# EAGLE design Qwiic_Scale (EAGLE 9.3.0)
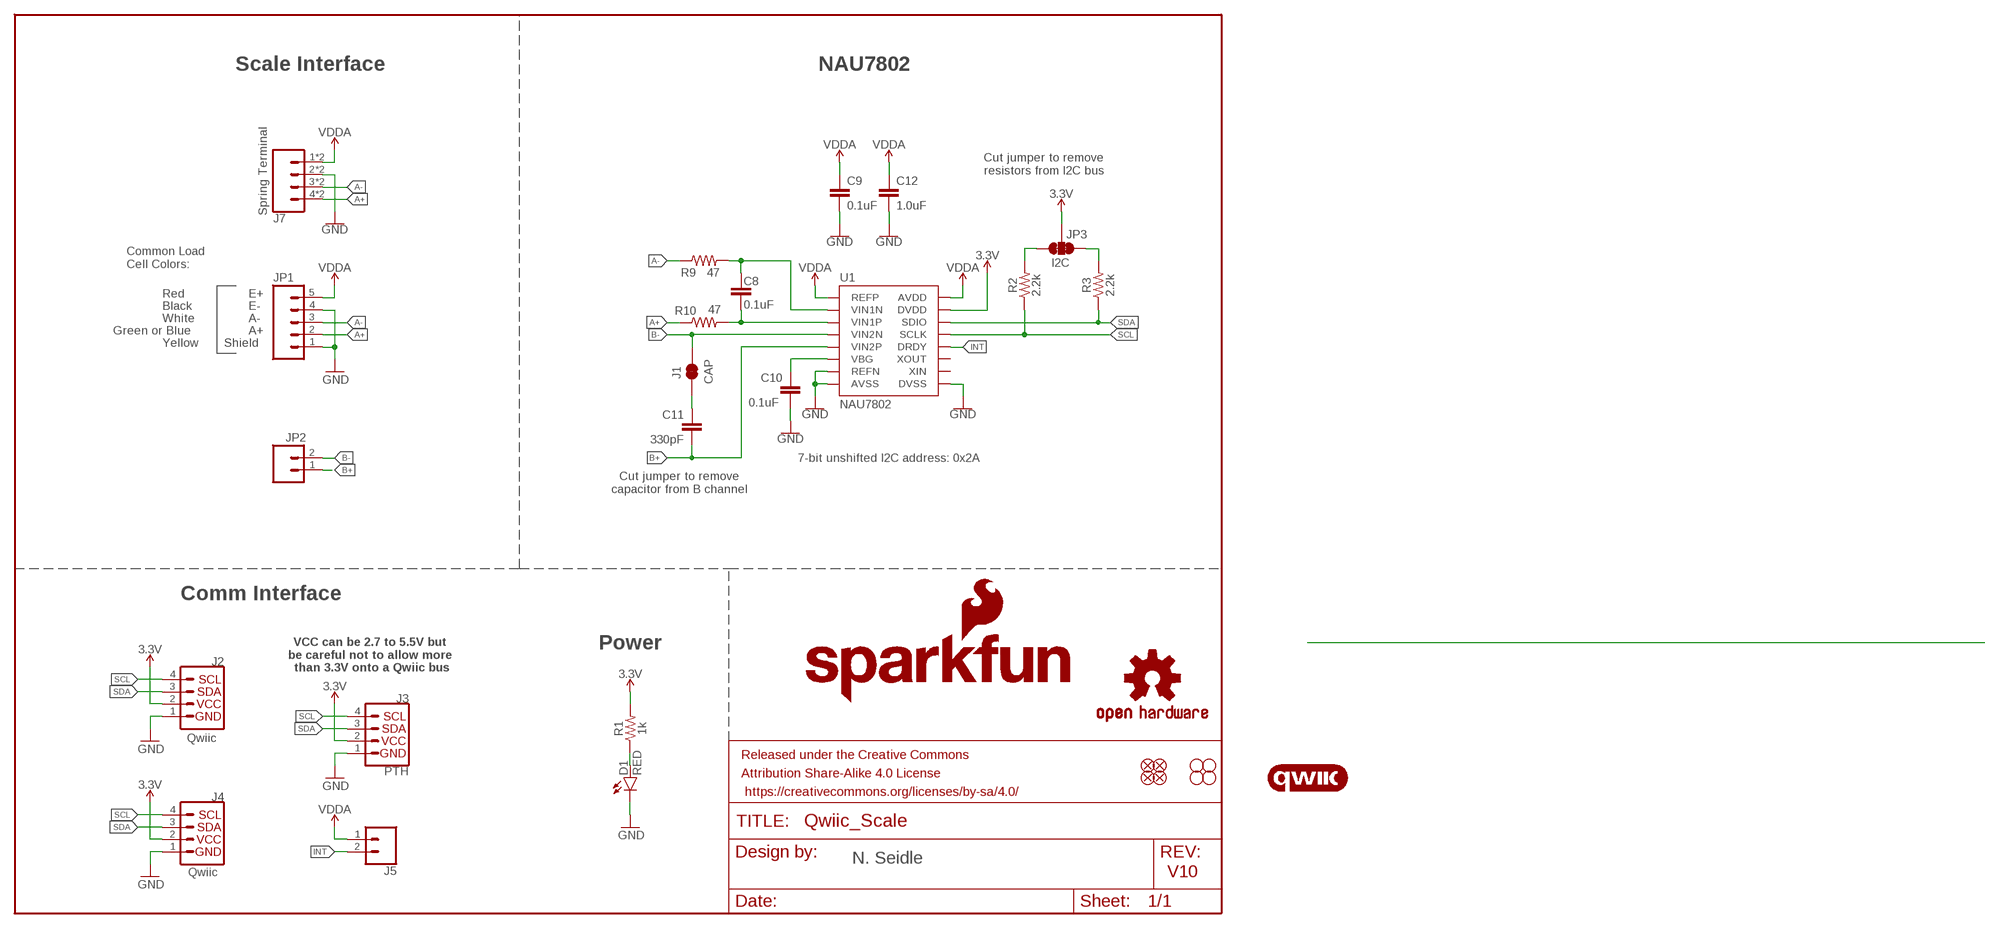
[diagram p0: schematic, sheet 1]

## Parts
C8  0.1uF  0.1UF-0603-25V-(+80/-20%)  [0603]
C9  0.1uF  0.1UF-0603-25V-(+80/-20%)  [0603]
C10  0.1uF  0.1UF-0603-25V-(+80/-20%)  [0603]
C11  330pF  330PF-0603-50V-5%  [0603]
C12  1.0uF  1.0UF-0603-16V-10%  [0603]
D1  RED  LED-RED0603  [LED-0603]
FRAME1  FRAME-LETTER  [CREATIVE_COMMONS]
J1  CAP  JUMPER-SMT_2_NC_TRACE_SILK  [SMT-JUMPER_2_NC_TRACE_SILK]
J2  Qwiic  I2C_STANDARDQWIIC  [JST04_1MM_RA]
J3  PTH  I2C_STANDARD_NO_SILK  [1X04_NO_SILK]
J4  Qwiic  I2C_STANDARDQWIIC  [JST04_1MM_RA]
J5  CONN_021X02_NO_SILK  [1X02_NO_SILK]
J7  Spring Terminal  CONN_04SPRING  [1X04_SPRING_TERMINAL]
JP1  CONN_05NO_SILK  [1X05_NO_SILK]
JP2  CONN_021X02_NO_SILK  [1X02_NO_SILK]
JP3  I2C  JUMPER-SMT_3_2-NC_TRACE_SILK  [SMT-JUMPER_3_2-NC_TRACE_SILK]
JP21  FIDUCIALUFIDUCIAL  [MICRO-FIDUCIAL]
JP31  STAND-OFF  [STAND-OFF]
JP41  STAND-OFF  [STAND-OFF]
JP61  FIDUCIALUFIDUCIAL  [MICRO-FIDUCIAL]
JP71  FIDUCIALUFIDUCIAL  [MICRO-FIDUCIAL]
JP81  FIDUCIALUFIDUCIAL  [MICRO-FIDUCIAL]
JP91  STAND-OFF  [STAND-OFF]
JP101  STAND-OFF  [STAND-OFF]
LOGO1  OSHW-LOGOMINI  [OSHW-LOGO-MINI]
LOGO2  SFE_LOGO_NAME_FLAME.1_INCH  [SFE_LOGO_NAME_FLAME_.1]
R1  1k  1KOHM-0603-1/10W-1%  [0603]
R2  2.2k  2.2KOHM-0603-1/10W-1%  [0603]
R3  2.2k  2.2KOHM-0603-1/10W-1%  [0603]
R9  47  47OHM-0603-1/10W-1%  [0603]
R10  47  47OHM-0603-1/10W-1%  [0603]
U1  NAU7802  NAU7802SOIC  [SO16]
U$26  QWIIC_LOGO_8MM  [QWIIC_8MM]

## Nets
3.3V [3.3V]: J2.2 J3.2 J4.2 JP3.2 R1.2 U1.15(DVDD)
A+: J7.4 J7.8 JP1.2 R10.1
A-: J7.3 J7.7 JP1.3 R9.1
B+: C11.2 JP2.1 U1.5(VIN2P)
B-: J1.2 JP2.2 U1.4(VIN2N)
GND: C9.2 C10.2 C12.2 D1.C J2.1 J3.1 J4.1 J7.2 J7.6 JP1.1 JP1.4 U1.7(REFN) U1.8(AVSS) U1.9(DVSS)
INT: J5.2 U1.12(DRDY)
N$1: C11.1 J1.1
N$2: JP3.1 R3.2
N$3: JP3.3 R2.2
N$10: D1.A R1.1
N$11: C10.1 U1.6(VBG)
N$15: C8.2 R10.2 U1.3(VIN1P)
N$16: C8.1 R9.2 U1.2(VIN1N)
SCL: J2.4 J3.4 J4.4 R2.1 U1.13(SCLK)
SDA: J2.3 J3.3 J4.3 R3.1 U1.14(SDIO)
VDDA: C9.1 C12.1 J5.1 J7.1 J7.5 JP1.5 U1.1(REFP) U1.16(AVDD)
Unconnected: U1.10(XIN) U1.11(XOUT)

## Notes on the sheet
- Scale Interface | NAU7802
- Cut jumper to remove
  resistors from I2C bus
- Common Load
  Cell Colors:
- Red | E+
- Black | E-
- White | A-
- Green or Blue | A+
- Yellow | Shield
- 7-bit unshifted I2C address: 0x2A
- Cut jumper to remove
  capacitor from B channel
- Comm Interface
- Power
- VCC can be 2.7 to 5.5V but 
  be careful not to allow more 
  than 3.3V onto a Qwiic bus
- N. Seidle
- V10

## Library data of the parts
C8-C10 = SparkFun-Capacitors:0.1UF: 0.1µF ceramic capacitors; PROD_ID: CAP-00810
C11 = SparkFun-Capacitors:330PF: 330pF/0.33nF ceramic capacitors; PROD_ID: CAP-10108
C12 = SparkFun-Capacitors:1.0UF: 1µF ceramic capacitors; PROD_ID: CAP-00868
D1 = SparkFun-LED:LED-RED: Red SMD LED; PROD_ID: DIO-00819
FRAME1 = SparkFun-Aesthetics:FRAME-LETTER: Schematic Frame - Letter
J1 = SparkFun-Jumpers:JUMPER-SMT_2_NC_TRACE: Normally closed trace jumper
J2 J4 = SparkFun-Connectors:I2C_STANDARD: SparkFun I2C Standard Pinout Header SparkFun has standardized on a pinout for all I2C based sensor breakouts. This pinout allows I2C boards to be plugged directly into the headers on Arduino Uno compatible boards, and to be daisy chained easily. Example SparkFun Products: SparkFun Atmospheric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; PROD_ID: CONN-13694; VALUE: Qwiic Right Angle
J3 = SparkFun-Connectors:I2C_STANDARD: SparkFun I2C Standard Pinout Header SparkFun has standardized on a pinout for all I2C based sensor breakouts. This pinout allows I2C boards to be plugged directly into the headers on Arduino Uno compatible boards, and to be daisy chained easily. Example SparkFun Products: SparkFun Atmospheric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
J5 JP2 = SparkFun-Connectors:CONN_02: Multi connection point. Often used as Generic Header-pin footprint for 0.1 inch spaced/style header connections
J7 = SparkFun-Connectors:CONN_04: Multi connection point. Often used as Generic Header-pin footprint for 0.1 inch spaced/style header connections On any of the 0.1 inch spaced packages, you can populate with these: Break Away Headers - Straight (PRT-00116) Break Away Male Headers - Right Angle (PRT-00553) Female Headers (PRT-00115)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; SF_ID: PRT-08075
JP1 = SparkFun-Connectors:CONN_05: Multi connection point. Often used as Generic Header-pin footprint for 0.1 inch spaced/style header connections On any of the 0.1 inch spaced packages, you can populate with these: Break Away Headers - Straight (PRT-00116) Break Away Male Headers - Right Angle (PRT-00553) Female Headers (PRT-00115)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
JP3 = SparkFun-Jumpers:JUMPER-SMT_3_2-NC_TRACE: Normally closed trace jumper (2 of 2 connections) This jumper has a trace between all three pads so they are normally closed (NC). Use a razor knife to open the connection(s). For best results follow the IPC guidelines for cutting traces: Cutout at least 0.063 mm (0.005 in). Remove all loose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
JP21 JP61 JP71 JP81 = SparkFun:FIDUCIAL: Fiducial Alignment Points
JP31 JP41 JP91 JP101 = SparkFun:STAND-OFF: Stand Off
LOGO1 = SparkFun-Aesthetics:OSHW-LOGO: Open-Source Hardware (OSHW) Logo
LOGO2 = SparkFun-Aesthetics:SFE_LOGO_NAME_FLAME: SparkFun Font Logo w/ Flame
R1 = SparkFun-Resistors:1KOHM: 1kΩ resistor; PROD_ID: RES-07856
R2 R3 = SparkFun-Resistors:2.2KOHM: 2.2kΩ resistor; PROD_ID: RES-08272
R9 R10 = SparkFun-Resistors:47OHM: 47Ω resistor; PROD_ID: RES-14282
U1 = SparkFun-IC-Conversion:NAU7802: 24-bit load cell conversion IC with I2C interface in SOIC-16 package. Similar to HX711 but with true I2C interface.; PROD_ID: IC-14299
U$26 = Qwiic_Logo:QWIIC_LOGO: Qwiic Logos for placement on schematic and PCB. The 5.5mm silk logo is best for placing next to Qwiic connector.

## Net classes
1 power: width 0.178 mm
2 3.3V: width 0.508 mm

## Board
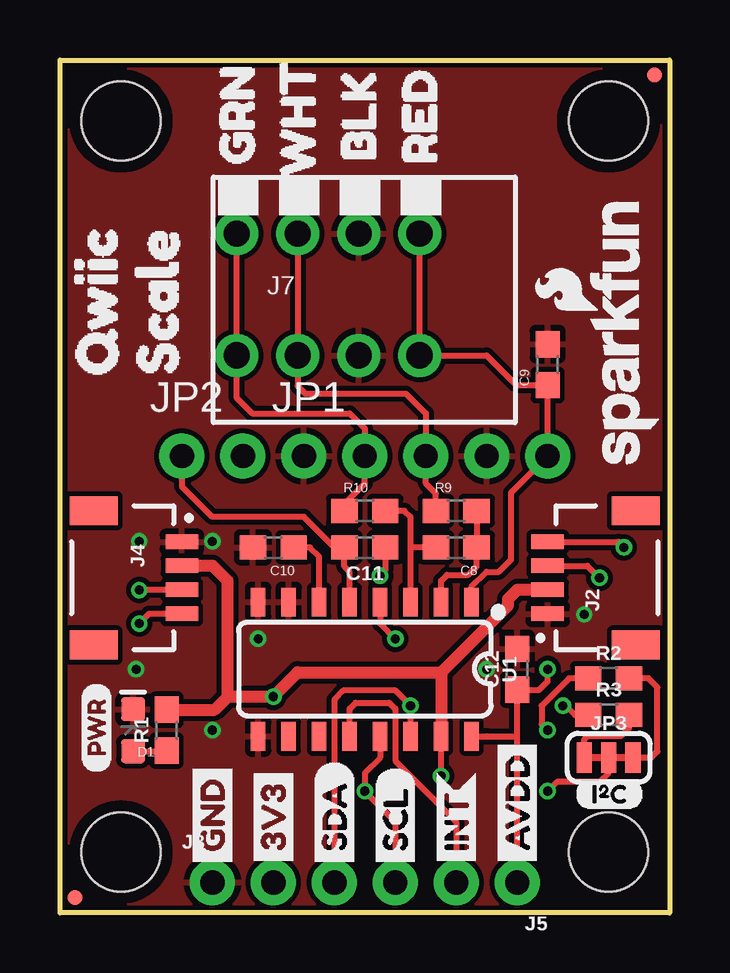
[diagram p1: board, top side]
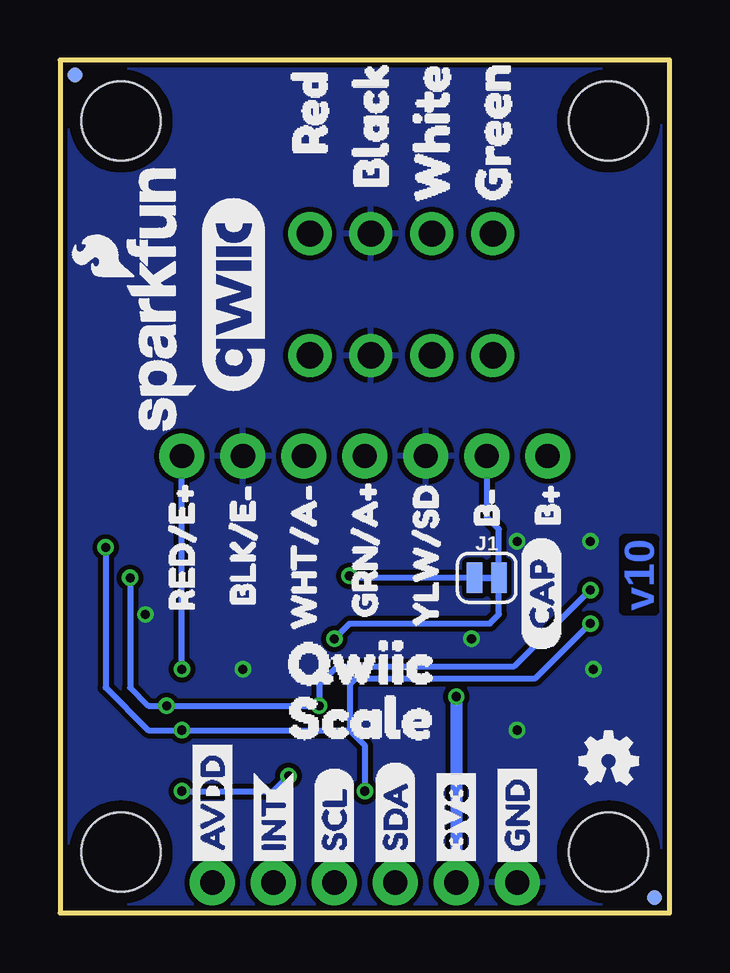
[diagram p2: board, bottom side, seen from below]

Size 25.4 x 35.56 mm. Coordinates in mm from the lower left corner, seen from the top.
Outline: 25.4,0 0,0 0,35.56 25.4,35.56 25.4,0
Copper layers (1*16): Top 0.035mm / dielectric 1.5mm / Bottom 0.035mm
Design rules "SparkFun-2-layer-PCBWay-LIMIT": minimum track width 6mil, minimum drill 0.3mm, track to track 6mil, track to pad 6mil, pad to pad 6mil, via to via 6mil, smd to smd 6mil, copper to edge 6mil, drill to drill 6mil, minimum pad ring 6mil, minimum via ring 6mil, stop-mask expansion 4mil, vias tented up to drill 25mil, thermal gap 10mil

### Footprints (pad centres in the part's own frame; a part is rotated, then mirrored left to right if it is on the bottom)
0603 = smd 1.1 x 1: 1 -0.85,0; 2 0.85,0
LED-0603 = smd 1 x 1: A -0.877,0; C 0.877,0
SMT-JUMPER_2_NC_TRACE_SILK = smd 0.635 x 1.27: 1 -0.508,0; 2 0.508,0
JST04_1MM_RA = smd 0.6 x 1.35: 1 -1.5,0; 2 -0.5,0; 3 0.5,0; 4 1.5,0 | smd 1.2 x 2: NC1 2.8,-3.675; NC2 -2.8,-3.675
1X04_NO_SILK = drill 1.016 pad 1.88: 1 0,0; 2 2.54,0; 3 5.08,0; 4 7.62,0
1X02_NO_SILK = drill 1.016 pad 1.88: 1 0,0; 2 2.54,0
1X04_SPRING_TERMINAL = drill 1.1 pad 1.8: 1 7.62,2.54; 2 5.08,2.54; 3 2.54,2.54; 4 0,2.54; 5 7.62,-2.54; 6 5.08,-2.54; 7 2.54,-2.54; 8 0,-2.54
1X05_NO_SILK = drill 1.016 pad 1.88: 1 0,0; 2 2.54,0; 3 5.08,0; 4 7.62,0; 5 10.16,0
SMT-JUMPER_3_2-NC_TRACE_SILK = smd 0.635 x 1.27: 1 -1.016,0; 2 0,0; 3 1.016,0
MICRO-FIDUCIAL = smd 0.635 x 0.635: 1 0,0
STAND-OFF = hole 3.302: 0,0
SO16 = smd 0.6 x 1.2: 1 -4.445,-2.8; 2 -3.175,-2.8; 3 -1.905,-2.8; 4 -0.635,-2.8; 5 0.635,-2.8; 6 1.905,-2.8; 7 3.175,-2.8; 8 4.445,-2.8; 9 4.445,2.8; 10 3.175,2.8; 11 1.905,2.8; 12 0.635,2.8; 13 -0.635,2.8; 14 -1.905,2.8; 15 -3.175,2.8; 16 -4.445,2.8

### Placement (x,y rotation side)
C8  16.51,15.24 180 top
C9  20.32,22.86 90 top
C10  8.89,15.24 180 top
C11  12.7,15.24 180 top
C12  19.05,10.16 90 top
D1  3.05,7.62 90 top
FRAME1  not placed on the board
J1  7.62,13.97 0 bottom
J2  20.32,13.97 90 top
J3  6.35,1.27 0 top
J4  5.08,13.97 270 top
J5  19.05,1.27 180 top
J7  7.37,25.78 0 top
JP1  10.16,19.05 0 top
JP2  5.08,19.05 0 top
JP3  22.86,6.48 0 top
JP21  24.77,34.92 90 top
JP31  2.54,2.54 90 top
JP41  2.54,33.02 90 top
JP61  0.64,0.64 90 top
JP71  24.77,34.92 270 bottom
JP81  0.64,0.64 270 bottom
JP91  22.86,2.54 90 top
JP101  22.86,33.02 90 top
LOGO1  2.54,6.35 0 bottom
LOGO2  21.21,25.65 90 bottom
LOGO3  SFE_LOGO_NAME_FLAME.1_INCH  [SFE_LOGO_NAME_FLAME_.1]  23.5,24.26 90 top
R1  4.45,7.62 90 top
R2  22.86,9.78 0 top
R3  22.86,8.26 0 top
R9  16.51,16.76 0 top
R10  12.7,16.76 0 top
U1  12.7,10.16 180 top
U$1  [SDA-[)]  11.43,1.65 90 top
U$3  [SCL-[)]  13.97,1.65 90 top
U$4  [SDA-[)]  11.43,1.65 90 bottom
U$5  [SCL-[)]  13.97,1.65 90 bottom
U$6  [3V3-04]  8.89,1.65 90 top
U$7  [3V3-04]  8.89,1.65 90 bottom
U$8  [GND-04]  6.35,1.65 90 top
U$9  [GND-04]  6.35,1.65 90 bottom
U$11  [YLW#SD4]  10.16,11.05 90 bottom
U$12  [B#11]  7.62,15.24 90 bottom
U$13  [B#12]  5.08,15.24 90 bottom
U$14  [QWIIC2]  17.4,10.41 0 bottom
U$15  [INT0]  16.51,1.65 90 bottom
U$17  [SCALE3]  17.4,8.13 0 bottom
U$18  [PWR-()-03]  1.52,5.84 90 top
U$19  [I_SUPER2_C-()-03]  21.46,4.95 0 top
U$20  [CAP0]  5.33,10.92 90 bottom
U$21  [INT0]  16.51,1.65 90 top
U$22  [QWIIC2]  1.52,20.95 90 top
U$24  [SCALE3]  4.06,20.95 90 top
U$26  18.16,25.78 90 bottom
U$34  [BLK#E#1]  17.78,11.94 90 bottom
U$35  [GRN#A#4]  12.7,11.43 90 bottom
U$36  [AVDD4]  19.05,1.65 90 top
U$37  [BLACK5]  12.45,28.96 90 bottom
U$38  [BLK1]  12.45,30.1 90 top
U$39  [GREEN7]  7.37,28.45 90 bottom
U$40  [GRN3]  7.37,29.97 90 top
U$41  [RED0]  14.99,29.97 90 top
U$42  [RED4]  14.99,30.35 90 bottom
U$43  [WHITE6]  9.91,28.19 90 bottom
U$44  [WHT2]  9.91,29.46 90 top
U$45  [AVDD4]  19.05,1.65 90 bottom
U$46  [RED#E#2]  20.32,11.68 90 bottom
U$48  [WHT#A#3]  15.24,10.92 90 bottom

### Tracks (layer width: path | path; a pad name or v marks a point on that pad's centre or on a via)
3.3V  (via drill 0.38)
  Top 0.254: JP3.2 22.86,5.84 22.48,5.46 20.7,5.46 v20.32,5.08 | v15.88,5.71 U1.15
  Top 0.508: 6.99,9.02 6.99,13.84 6.36,14.47 J4.2 | J2.2 19.06,13.47 18.67,13.08 18.67,12.83 15.88,10.03 | 15.88,10.03 U1.15 | 6.99,9.02 v8.89,9.02 9.91,10.03 15.88,10.03 | 6.99,9.02 6.44,8.47 R1.2
  Bottom 0.254: v20.32,5.08 16.51,5.08 v15.88,5.71
  Bottom 0.508: v8.89,9.02 J3.2
A+
  Top 0.254: R10.1 11.85,17.06 12.7,17.91 JP1.2 12.7,20.19 12.06,20.83 8,20.83 7.37,21.46 J7.8 J7.4
A-
  Top 0.254: J7.3 J7.7 9.91,21.97 10.22,21.65 14.41,21.65 15.24,20.83 JP1.3 15.24,17.91 15.66,17.49 R9.1
B+
  Top 0.254: U1.5 12.06,14.22 11.85,14.44 C11.2 11.43,15.24 10.16,16.51 6.35,16.51 5.08,17.78 JP2.1
B-  (via drill 0.38)
  Top 0.254: U1.4 13.34,12.06 v13.97,11.43
  Bottom 0.254: v13.97,11.43 13.34,12.06 7.49,12.06 7.11,12.45 J1.2 7.11,16 7.62,16.51 JP2.2
GND  (via drill 0.38)
  other vias: 17.78,10.16 6.35,7.62 3.17,10.16 3.3,15.49 21.84,12.45 6.35,15.49 8.26,11.43
  pour Top (isolate 0.203, rank 4): 0,0 0,35.56 25.4,35.56 25.4,0
  pour Bottom (isolate 0.203, rank 4): 0,0 0,35.56 25.4,35.56 25.4,0
INT
  Top 0.254: U1.12 12.06,8.51 12.32,8.76 13.72,8.76 13.97,8.51 13.97,6.35 16.51,3.81 J5.2
N$1  (via drill 0.38)
  Top 0.254: C11.1 13.55,14.27 v13.34,14.05
  Bottom 0.254: v13.34,14.05 13.25,13.97 J1.1
N$2
  Top 0.254: JP3.1 21.84,7.24 22,7.39 23.39,7.39 23.71,7.71 R3.2
N$3
  Top 0.254: JP3.3 24.64,6.48 24.89,6.73 24.89,9.4 24.51,9.78 R2.2
N$10
  Top 0.254: D1.A 4.42,6.74 R1.1
N$11
  Top 0.254: U1.6 10.79,14.86 10.41,15.24 C10.1
N$15
  Top 0.254: U1.3 14.61,15.24 | 14.61,15.24 14.61,16.51 14.35,16.76 R10.2 | C8.2 14.61,15.24
N$16
  Top 0.254: R9.2 C8.1 17.36,14.44 17.02,14.1 16.13,14.1 15.88,13.84 U1.2
SCL  (via drill 0.38)
  Top 0.254: U1.13 13.34,6.47 12.7,5.84 v12.7,5.08 13.97,3.81 J3.4 | J2.4 23.27,15.47 v23.5,15.24 | J4.4 3.71,12.47 v3.3,12.06 | R2.1 21.21,9.78 20.07,8.64 20.07,7.87 v20.32,7.62
  Bottom 0.254: v23.5,15.24 23.5,9.4 21.72,7.62 v20.32,7.62 13.34,7.62 | v3.3,12.06 5.59,9.78 13.08,9.78 13.34,9.53 13.34,7.62 | 13.34,7.62 12.7,6.99 v12.7,5.08
SDA  (via drill 0.38)
  Top 0.254: U1.14 v14.61,8.64 13.97,9.27 11.81,9.27 11.43,8.89 J3.3 | J2.3 21.98,14.47 v22.48,13.97 | J4.3 v3.31,13.47 v3.3,13.46 | R3.1 21.46,8.26 21.08,8.64 v20.95,8.64
  Bottom 0.254: v22.48,13.97 22.48,9.4 21.72,8.64 v20.95,8.64 v14.61,8.64 14.61,9.53 13.84,10.29 6.48,10.29 v3.3,13.46
VDDA  (via drill 0.38)
  Top 0.254: U1.16 17.78,7.36 17.79,7.37 19.05,7.37 | U1.1 17.14,13.59 17.78,14.22 18.29,14.22 18.8,14.73 18.8,17.53 JP1.5 C9.1 19.01,22.01 17.78,23.24 J7.5 J7.1 | J5.1 19.05,7.37 | 19.05,7.37 C12.1 19.98,9.31 20.32,9.65 v20.32,10.16
  Bottom 0.254: v20.32,10.16 JP1.5

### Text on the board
Bottom: v10
Measures: Units in inches
tDocu: N. Seidle

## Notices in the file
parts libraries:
SparkFun-Resistors: Licensing: Creative Commons ShareAlike 4.0 International - https://creativecommons.org/licenses/by-sa/4.0
SparkFun-Aesthetics: Released under the Creative Commons Attribution Share-Alike 4.0 License
SparkFun-Aesthetics: https://creativecommons.org/licenses/by-sa/4.0
